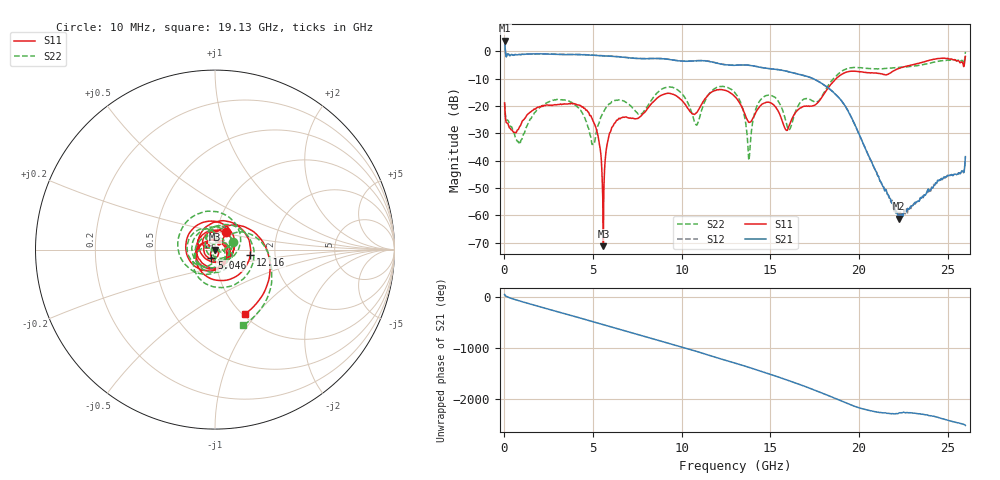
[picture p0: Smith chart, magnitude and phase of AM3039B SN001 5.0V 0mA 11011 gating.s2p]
!Agilent Technologies,E8364B,MY43040894,A.07.50.67
!Agilent E8364B: A.07.50.67
!Date: Tuesday, June 28, 2016 08:12:35
!Correction: S11(Full 2 Port(1,2))
!S21(Full 2 Port(1,2))
!S12(Full 2 Port(1,2))
!S22(Full 2 Port(1,2))
!S2P File: Measurements: S11, S21, S12, S22:
# Hz S  dB  R 50
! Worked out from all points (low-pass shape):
!   1601 points, 10 MHz to 26 GHz, reference 50 ohm
!   highest |S21| = 3.84 dB at 10 MHz (marker M1); lowest = -61.2 dB at 22.25 GHz (marker M2)
!   |S21| within 3 dB of the highest: start of sweep to 43.92 MHz
!   lowest |S11| = -71.3 dB at 5.582 GHz (marker M3), VSWR 1.00, Z = 50 - j0.00869 ohm
!   |S11| at or under -10 dB: start of sweep to 18.72 GHz
!   |S22| runs from -39.9 to -0.3 dB; largest |S21 - S12| = 0.025
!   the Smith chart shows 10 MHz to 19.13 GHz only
!   S11 on the Smith chart (normalised r, x): 10 MHz: 1.10, +0.22; 5.046 GHz: 0.96, -0.09; 12.16 GHz: 1.48, -0.09; 19.13 GHz: 1.03, -0.87
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1e7  -18.91 58.3  3.84 41.1  3.91 41.9  -19.17 22.3
7.572125e8  -28.72 58.8  -1.30 -73.5  -1.25 -73.3  -33.12 -14.9
1.764325e9  -21.03 -19.5  -1.02 -174.4  -0.98 -174.3  -22.11 -49.2
2.852656e9  -19.54 -167.4  -1.14 79.8  -1.11 80.0  -17.74 174.3
4.347081e9  -20.35 -20.2  -1.29 -64.5  -1.26 -64.5  -22.15 -25.5
5.045562e9  -26.12 -113.3  -1.51 -133.4  -1.46 -133.3  -33.79 137.6
5.581606e9  -71.29 -18.6  -1.73 174.0  -1.68 174.1  -22.36 16.8
6.410038e9  -24.99 -116.9  -2.05 92.1  -2.00 92.0  -17.88 -99.6
7.2872e9  -24.63 102.0  -2.61 6.1  -2.57 6.1  -21.18 124.6
8.684162e9  -16.80 -139.0  -2.68 -131.3  -2.62 -131.3  -14.88 -148.1
1.003239e10  -18.17 29.4  -3.68 93.0  -3.62 92.9  -15.73 30.6
1.102326e10  -20.54 168.8  -3.47 -7.1  -3.41 -7.4  -23.90 148.6
1.216032e10  -14.06 -8.3  -4.63 -128.7  -4.61 -129.0  -12.95 -26.4
1.3005e10  -16.63 -118.7  -5.16 146.7  -5.13 146.3  -15.25 -126.5
1.380094e10  -26.04 74.0  -5.15 58.9  -5.11 58.6  -39.68 -131.0
1.503547e10  -19.00 -159.4  -6.48 -78.9  -6.45 -79.3  -16.16 154.8
1.734208e10  -20.09 87.6  -9.86 -2.2  -9.87 -2.7  -18.08 48.0
1.912889e10  -8.08 -64.6  -19.19 106.5  -19.19 106.2  -6.95 -69.7
2.167916e10  -8.28 53.7  -52.84 -117.9  -53.40 -119.6  -6.27 59.0
2.224769e10  -6.31 9.9  -61.22 -111.5  -58.78 -116.9  -5.95 14.5
2.461928e10  -2.58 176.4  -46.87 149.0  -46.69 146.5  -3.53 -167.0
2.6e10  -1.92 13.5  -38.56 8.1  -38.70 7.5  -0.25 46.6
